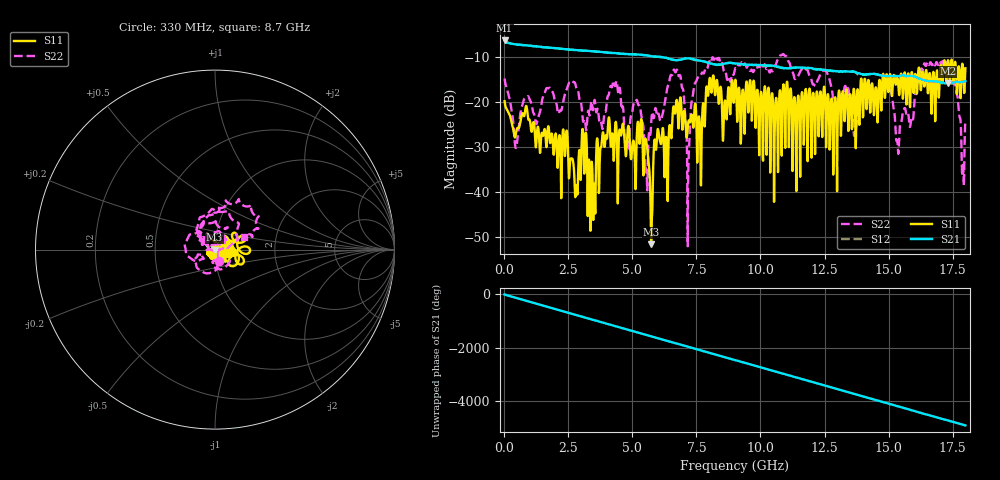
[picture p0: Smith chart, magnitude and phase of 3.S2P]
!Agilent Technologies,E5071C,MY46316741,A.11.02
!Date: Thu Sep 29 15:36:59 2022
!Data & Calibration Information:
!Freq	S11:SOLT2(ON)	S21:SOLT2(ON)	S12:SOLT2(ON)	S22:SOLT2(ON)
!PortZ  Port1:50+j0  Port2:50+j0
!Above PortZ is port z conversion or system Z0 setting when saving the data.
!When reading, reference impedance value at option line is always used.
# Hz S dB R 50
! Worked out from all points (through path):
!   1800 points, 10 MHz to 18 GHz, reference 50 ohm
!   highest |S21| = -6.42 dB at 10 MHz (marker M1); lowest = -15.9 dB at 17.31 GHz (marker M2)
!   group delay of S21, straight-line fit = 757 ps
!   lowest |S11| = -51.5 dB at 5.73 GHz (marker M3), VSWR 1.01, Z = 49.7 - j0.0558 ohm
!   |S11| at or under -10 dB: start of sweep to end of sweep
!   |S22| runs from -52.0 to -9.4 dB; largest |S21 - S12| = 0.02
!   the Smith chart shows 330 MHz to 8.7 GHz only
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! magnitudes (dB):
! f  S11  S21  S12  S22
! 10 MHz  -19.9  -6.4  -6.4  -14.9
! 460 MHz  -26.7  -7.3  -7.3  -30.2
! 860 MHz  -20.9  -7.5  -7.5  -19.1
! 2.79 GHz  -39.9  -8.6  -8.6  -16.5
! 3.01 GHz  -30.5  -8.6  -8.6  -20.8
! 3.44 GHz  -36.2  -8.8  -8.8  -21.3
! 4.04 GHz  -26.0  -9.1  -9.1  -18.7
! 4.79 GHz  -28.3  -9.5  -9.5  -30.6
! 5.29 GHz  -28.8  -9.6  -9.5  -21.0
! 5.54 GHz  -28.8  -9.7  -9.7  -34.8
! 5.73 GHz  -51.5  -9.9  -9.9  -25.1
! 6.01 GHz  -26.3  -10.0  -10.0  -22.6
! 6.79 GHz  -25.3  -10.8  -10.7  -14.0
! 7.17 GHz  -25.2  -10.4  -10.4  -40.0
! 7.52 GHz  -31.1  -10.8  -10.8  -15.0
! 9.01 GHz  -15.3  -11.5  -11.5  -12.7
! 12.01 GHz  -24.4  -12.6  -12.6  -15.6
! 13.7 GHz  -24.1  -13.4  -13.4  -26.7
! 15.01 GHz  -16.8  -14.3  -14.3  -16.1
! 15.36 GHz  -15.0  -14.3  -14.3  -29.9
! 17.31 GHz  -11.0  -15.9  -16.0  -12.5
! 18 GHz  -12.6  -15.5  -15.6  -24.0
